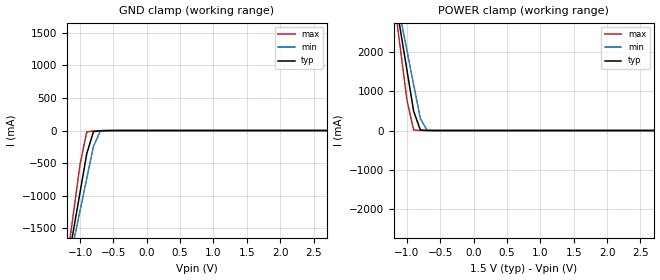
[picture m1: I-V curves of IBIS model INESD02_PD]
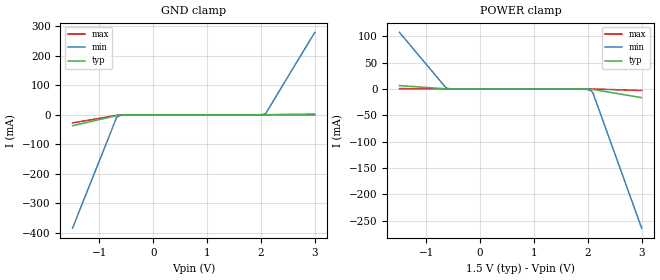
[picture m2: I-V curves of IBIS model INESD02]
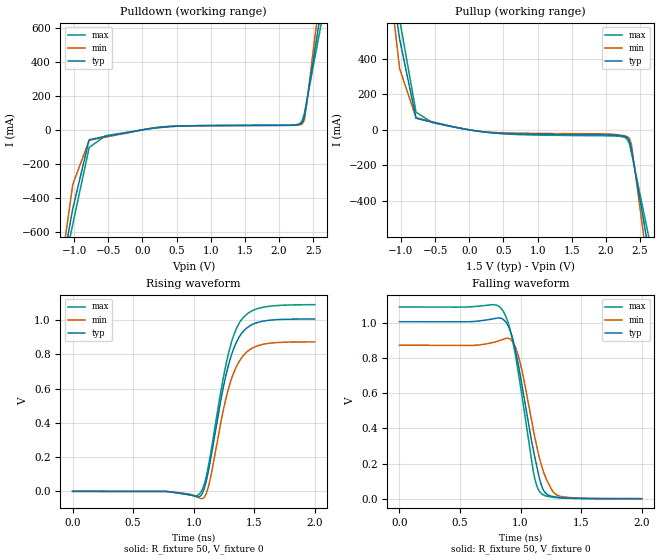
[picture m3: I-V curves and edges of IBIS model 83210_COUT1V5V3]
|   This file is an IBIS representation of the   |
|   Integrated Device Technology , Inc.   |
|   ICS83210   |
|   Low Skew 1 to 10  HSTL Fanout Buffer   |
[IBIS Ver]   4.1
[File name]   83210_1v5.ibs
[File Rev]   1.0
[Date]   28 Aug 2009 | Last modified
|   Aug 30 2001 | Generated
[Source]   Originated at Integrated Device Technology, Inc.
[Disclaimer]
IDT hereby grants the user of this IBIS model a non-exclusive,
nontransferable license to use this IBIS model under the following terms.
Before using this IBIS model, the user should read this license.
If the user does not accept these terms,  the IBIS model should be
returned to IDT within 30 days.
   The user is granted this license only to use the IBIS model and
is not granted rights to sell, load, rent, lease or license the IBIS
model in whole or in part, or in modified form to anyone other than
user. User may modify the IBIS model to suit its specific
applications but rights to derivative works and such modifications
shall belong to IDT.
   This IBIS model is provided on an "AS IS" basis and IDT makes
absolutely no warranty with respect to the information contained
herein. IDT DISCLAIMS AND CUSTOMER WAIVES ALL WARRANTIES, EXPRESS
OR IMPLIED, INCLUDING WARRANTIES OF MERCHANTABILITY OR FITNESS FOR
A PARTICULAR PURPOSE. The entire risk as to quality and performance
is with the Customer. ACCORDINGLY, IN NO EVENT SHALL THE COMPANY BE
LIABLE FOR ANY DAMAGES, WHETHER IN CONTRACT OR TORT,INCLUDING ANY
LOST PROFITS OR OTHER INCIDENTAL, CONSEQUENTIAL, EXEMPLARY, OR
PUNITIVE DAMAGES ARISING OUT OF THE USE OR APPLICATION OF THE IBIS
model provided in this package. Further, IDT reserves the right to
make changes without notice to any product herein to improve
reliability, function, or design. IDT does not convey any license
under patent rights or any other intellectual property rights,
including those of third parties.
   IDT is not obligated to provide maintenance or support
for the licensed IBIS model.
[Copyright]   Copyright 2005 by Integrated Device Technology , Inc.
[Component]   ICS83210Y
[Manufacturer] Integrated Device Technology, Inc.
[Package]
|TQFP32
|lead + wire   typ   min   max
R_pkg   86.05m   81.2m   90.9m
L_pkg   2.653n   2.410n   2.895n
C_pkg   0.407p   0.381p   0.433p   |
[Pin] signal_name   model_name   R_pin   L_pin   C_pin
1   VDD   POWER   238m   1.974n   0.330p
2   GND   GND   225m   1.841n   0.311p
3   VDD   POWER   218m   1.7745n   0.301p
4   nOE   INESD02_PD   213m   1.708n   0.291p
5   GND   GND   213m   1.708n   0.291p
6   IN   INESD02   218m   1.7745n   0.301p
7   VDD   POWER   225m   1.841n   0.311p
8   GND   GND   238m   1.974n   0.330p
9   GND   GND   238m   1.974n   0.330p
10   GND   GND   225m   1.841n   0.311p
11   Q9   83210_COUT1V5V3   218m   1.7745n   0.301p
12   VDD   POWER   213m   1.708n   0.291p
13   VDD   POWER   213m   1.708n   0.291p
14   Q8   83210_COUT1V5V3   218m   1.7745n   0.301p
15   Q7   83210_COUT1V5V3   225m   1.841n   0.311p
16   GND   GND   238m   1.974n   0.330p
17   GND   GND   238m   1.974n   0.330p
18   Q6   83210_COUT1V5V3   225m   1.841n   0.311p
19   Q5   83210_COUT1V5V3   218m   1.7745n   0.301p
20   VDD   POWER   213m   1.708n   0.291p
21   VDD   POWER   213m   1.708n   0.291p
22   Q4   83210_COUT1V5V3   218m   1.7745n   0.301p
23   Q3   83210_COUT1V5V3   225m   1.841n   0.311p
24   GND   GND   238m   1.974n   0.330p
25   GND   GND   238m   1.974n   0.330p
26   Q2   83210_COUT1V5V3   225m   1.841n   0.311p
27   Q1   83210_COUT1V5V3   218m   1.7745n   0.301p
28   VDD   POWER   213m   1.708n   0.291p
29   VDD   POWER   213m   1.708n   0.291p
30   Q0   83210_COUT1V5V3   218m   1.7745n   0.301p
31   GND   GND   225m   1.841n   0.311p
32   GND   GND   238m   1.974n   0.330p
| Models and submodels in the file (3): INESD02_PD (Input), INESD02 (Input), 83210_COUT1V5V3 (Output)
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[Model]   INESD02_PD
Model_type   Input
Polarity   Non-Inverting
Vinl = 0.45V
Vinh = 1.05V
|   typ   min   max
C_comp   2pF   1.5pF   2.5pF
|   typ   min   max
[Voltage range]   1.5V   1.425V   1.575V
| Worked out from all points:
|   GND clamp passes 1 mA (typ) near -0.60 V on its own axis
|   POWER clamp passes 1 mA (typ) near -0.70 V on its own axis
[GND_clamp]
|Voltage   I (typ)   I (min)   I (max)
-3.3V     -14.52A    -12.54A    -17.85A
-1.2V     -2.123A    -2.208A    -2.021A
-900mV    -353.5mA   -734.3mA   -21.76mA
-700mV    -3.491mA   -14.25mA   -2.553mA
3.8V      83.75uA    4.893mA    57.37uA
3.9V      169.7uA    99.2mA     58.9uA
4.1V      14.27mA    1.722A     76.17uA
4.3V      1.523A     3.446A     1.452mA
4.4V      2.557A     4.308A     69.84mA
4.5V      3.592A     5.171A     1.225A
4.6V      4.628A     6.034A     2.547A
6.6V      25.37A     23.32A     29.05A
[Power_clamp]
|Voltage   I (typ)   I (min)   I (max)
-3.3V     25.37A     21.89A     31.23A
-1.2V     3.592A     3.748A     3.407A
-1.1V     2.557A     2.885A     2.084A
-900mV    488.5mA    1.162A     13.85mA
-700mV    862uA      13.32mA    132.7uA
3.8V      -180.1uA   -6.224mA   -5.27uA
4.1V      -17.79mA   -1.053A    -1.005mA
4.3V      -943mA     -2.036A    -8.439mA
4.4V      -1.533A    -2.528A    -72.78mA
4.6V      -2.713A    -3.512A    -1.531A
4.8V      -3.894A    -4.496A    -3.039A
6.6V      -14.52A    -13.36A    -16.61A
[Model]   INESD02
Model_type   Input
Polarity   Non-Inverting
Vinl = 0.45V
Vinh = 1.05V
|   typ   min   max
C_comp   2pF   1.5pF   2.5pF
|   typ   min   max
[Voltage range]   1.5V   1.425V   1.575V
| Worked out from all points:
|   GND clamp passes 1 mA (typ) near -0.60 V on its own axis
|   POWER clamp passes 1 mA (typ) near -0.75 V on its own axis
[GND_clamp]
|Voltage   I (typ)   I (min)   I (max)
-1.5V     -37.09mA   -383.8mA   -27.55mA
-681.8mV  -2.849mA   -9.078mA   -2.022mA
-636.4mV  -1.676mA   -3.51mA    -1.019mA
-500mV    -170.4uA   -370.6uA   -50.37uA
1.909V    927.3nA    70.81uA    526.6pA
2.045V    28.17uA    1.479mA    87.56nA
2.091V    77.06uA    4.924mA    420.7nA
3V        2.572mA    279mA      28.1uA
[Power_clamp]
|Voltage   I (typ)   I (min)   I (max)
-1.5V     6.332mA    107.3mA    598.8uA
-636.4mV  201.8uA    2.218mA    14.78uA
-590.9mV  77.06uA    727.2uA    4.319uA
1.864V    -6.153uA   -116.5uA   -32.11nA
2V        -170.4uA   -1.27mA    -5.636uA
2.045V    -415.4uA   -2.647mA   -22.48uA
2.091V    -890.7uA   -6.331mA   -75.92uA
3V        -16.6mA    -264.1mA   -3.088mA
[Model]   83210_COUT1V5V3
Model_type   Output
Polarity   Non-Inverting
|   typ   min   max
C_comp   2pF   1.5pF   2.5pF
Vmeas = 0.5V
Rref = 50
Cref = 0
Vref = 0V
|   typ   min   max
[Voltage range]   1.5V   1.425V   1.575V
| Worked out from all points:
|   slope of the pulldown table from 0 to 0.225 V, typ, clamps not added: 17 ohm
|   slope of the pullup table from 0 to 0.225 V, typ, clamps not added: 18.7 ohm
|   rising waveform, R_fixture 50, V_fixture 0: 20-80 % time 173ps typ, 169ps min, 173ps max; typ from 0 V to 1.01 V
|   falling waveform, R_fixture 50, V_fixture 0: 20-80 % time 159ps typ, 158ps min, 148ps max; typ from 1.01 V to 0 V
[Pulldown]
|Voltage   I (typ)   I (min)   I (max)
-1.5V     -1.549A    -1.699A    -1.465A
-1.26V    -1.007A    -1.011A    -1.012A
-1.02V    -465mA     -322.8mA   -557.7mA
-780mV    -58.28mA   -61.6mA    -104.2mA
-540mV    -38.22mA   -42.78mA   -34.86mA
159mV     10mA       11.42mA    9.025mA
2.211V    27.72mA    26.77mA    28.79mA
2.34V     44.38mA    35.25mA    54.3mA
2.372V    80.71mA    59.79mA    98.04mA
2.51V     434.5mA    498.3mA    394.7mA
2.608V    687.6mA    821.6mA    605.7mA
3V        1.705A     2.12A      1.454A
[Pullup]
|Voltage   I (typ)   I (min)   I (max)
-1.5V     1.772A     1.948A     1.675A
-1.26V    1.141A     1.146A     1.147A
-1.02V    509.6mA    343.2mA    619.3mA
-780mV    65.23mA    68.25mA    99.13mA
-540mV    42.44mA    45.06mA    40.43mA
191mV     -10.51mA   -9.864mA   -10.73mA
2.308V    -42.93mA   -37.07mA   -50.97mA
2.34V     -58.3mA    -45.58mA   -72.76mA
2.372V    -106.8mA   -79.45mA   -124.7mA
2.51V     -416.2mA   -471.5mA   -382.3mA
2.608V    -635.9mA   -751.8mA   -565.4mA
3V        -1.517A    -1.874A    -1.301A
[Ramp]
|   typ   min   max
dV/dt_r   0.831/0.269n   0.732/0.268n   0.892/0.269n
dV/dt_f   0.822/0.232n   0.73/0.248n   0.883/0.218n
R_load =   50.0000
[Rising Waveform]
R_fixture = 50
V_fixture = 0
V_fixture_max = 0
V_fixture_min = 0
C_fixture = 0.0p
| Time   typ   min   max
0s        172.8pV    19.15pV    20.59nV
760.8ps   98.42uV    12.79uV    -30.68uV
1.041ns   -32.1mV    -36.76mV   -18.59mV
1.077ns   -2.419mV   -40.88mV   20.76mV
1.115ns   95.43mV    10.93mV    123.2mV
1.271ns   691.8mV    556mV      755.7mV
1.323ns   819.7mV    678.5mV    896.1mV
1.379ns   905.2mV    762.5mV    986.2mV
1.558ns   991.9mV    856.3mV    1.073V
2ns       1.007V     873mV      1.09V
[Falling Waveform]
R_fixture = 50
V_fixture = 0
V_fixture_max = 0
V_fixture_min = 0
C_fixture = 0.0p
| Time   typ   min   max
0s        1.007V     873.1mV    1.091V
826.8ps   1.028V     899.2mV    1.091V
900.9ps   977.6mV    911.9mV    993.8mV
969ps     808.3mV    840.9mV    771.2mV
1.019ns   615.5mV    706.2mV    551.8mV
1.103ns   285.1mV    401.2mV    164.1mV
1.159ns   107.7mV    223.3mV    39.16mV
1.209ns   30.1mV     117.7mV    15.62mV
1.311ns   7.613mV    17.23mV    5.169mV
2ns       7.428uV    17.11uV    5.675uV
